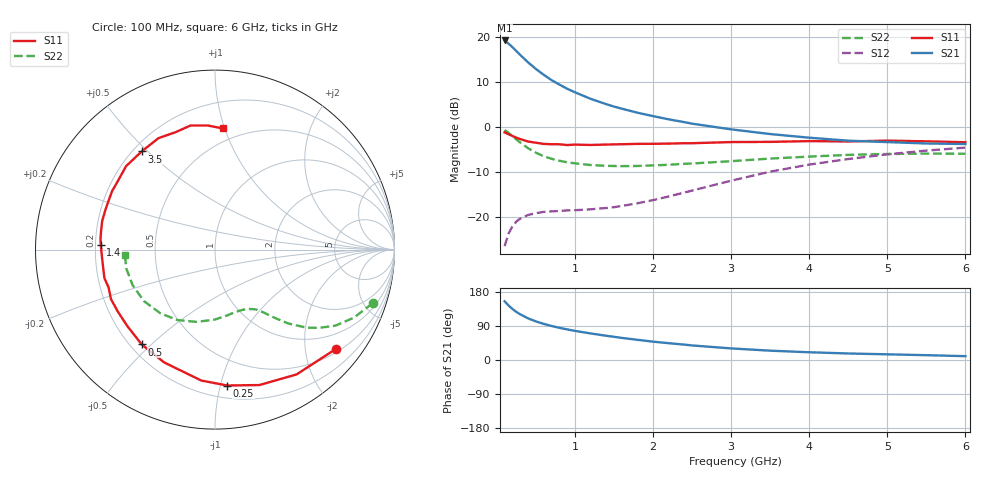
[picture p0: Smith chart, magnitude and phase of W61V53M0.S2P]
! SIEMENS Small Signal Semiconductors
! BFR193W
! Si NPN RF Bipolar Junction Transistor in SOT323
! VCE = 1.5 V  IC = 3 mA
! Common Emitter S-Parameters:  September  1992
# GHz  S  MA  R  50
!  f  S11  S21  S12  S22
! GHz  MAG  ANG  MAG  ANG  MAG  ANG  MAG  ANG
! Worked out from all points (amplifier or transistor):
!   28 points, 100 MHz to 6 GHz, reference 50 ohm
!   highest |S21| = 19.3 dB at 100 MHz (marker M1)
!   |S21| within 3 dB of that: start of sweep to 286.5 MHz
!   unconditionally stable (mu >= 1): 1.352 GHz to 2.656 GHz
!   at 300 MHz: K = 0.26, MSG = 18.3 dB, |S12| = -20.4 dB
!   at 1.5 GHz: K = 1.06, MAG = 9.8 dB, |S12| = -17.9 dB
!   at 6 GHz: K = 0.96, MSG = 0.4 dB, |S12| = -4.6 dB
!   S11 on the Smith chart (normalised r, x): 100 MHz: 0.58, -2.68; 250 MHz: 0.29, -1.05; 500 MHz: 0.24, -0.47; 1.4 GHz: 0.22, +0.02; 3.5 GHz: 0.23, +0.48; 6 GHz: 0.40, +0.98
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0.1  0.8718 -39.4  9.249 154.9  0.0468 68.9  0.9281 -18.8
0.15  0.8309 -56.8  8.525 144.0  0.0645 60.6  0.861 -26.2
0.2  0.7943 -71.8  7.788 134.7  0.0779 53.7  0.793 -32.3
0.25  0.7602 -84.9  7.044 127.0  0.0881 48.1  0.7261 -36.9
0.3  0.7334 -96.0  6.374 120.5  0.095 43.9  0.6714 -40.4
0.4  0.6895 -114.2  5.269 109.9  0.1043 38.0  0.5803 -45.2
0.5  0.6678 -127.7  4.448 101.9  0.1093 34.5  0.5171 -48.2
0.6  0.6485 -138.6  3.831 95.4  0.1129 32.7  0.4726 -50.6
0.7  0.6423 -147.3  3.342 89.8  0.1143 31.9  0.4424 -52.3
0.8  0.6419 -154.5  2.98 85.0  0.1157 32.0  0.4204 -54.2
0.9  0.6291 -160.4  2.677 80.8  0.1172 32.6  0.4039 -55.6
1  0.6364 -165.6  2.444 76.8  0.1179 33.7  0.3932 -57.5
1.2  0.6306 -174.8  2.066 70.1  0.1206 36.8  0.3765 -61.4
1.4  0.637 177.7  1.8 64.0  0.1248 40.9  0.369 -65.5
1.8  0.6485 165.8  1.445 53.3  0.1408 50.2  0.3676 -74.7
2.2  0.653 154.8  1.219 44.4  0.1679 57.4  0.3789 -84.2
2.5  0.6595 148.1  1.09 38.4  0.1953 60.8  0.3917 -91.5
3  0.6793 136.8  0.942 30.6  0.2516 62.7  0.4156 -104.4
3.5  0.6826 126.8  0.835 24.6  0.3175 60.5  0.4447 -118.0
4.5  0.6902 108.4  0.704 17.2  0.4395 51.0  0.489 -144.1
5.5  0.6922 93.2  0.655 12.7  0.5455 39.6  0.505 -167.9
6  0.6764 86.4  0.646 10.1  0.5892 33.3  0.5031 -176.8
